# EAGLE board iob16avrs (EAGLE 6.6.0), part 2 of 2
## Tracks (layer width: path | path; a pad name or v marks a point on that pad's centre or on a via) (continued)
GND  (via drill 0.38) (continued)
  Top 0.254: 23.74,28.91 23.7,28.87 23.7,28.3 23.74,28.26 24.49,28.26 CF1.15 | 23.74,28.91 CF1.39 | 23.74,28.91 23.7,29.02 23.7,29.51 23.74,29.55 24.49,29.55 CF1.14 26.43,29.55 v27.04,29.55 | IC12.110 87.69,56.53 86.89,56.53 86.86,56.57 86.86,56.98 86.89,57.02 87.69,57.02 IC12.109 89.26,57.02 v89.87,57.02 | v87.05,40.03 87.69,40.03 IC12.143 | v93.83,39.08 93.83,38.47 IC12.8 | v87.05,44.03 87.69,44.03 IC12.135 | v89.87,47.54 89.26,47.54 IC12.128 | v98.32,39.08 98.32,38.47 IC12.17 | v87.05,52.03 87.69,52.03 IC12.119 | v102.32,39.08 102.32,38.47 IC12.25 | v106.32,39.08 106.32,38.47 IC12.33 | v91.35,57.48 91.35,58.09 IC12.106 | v95.35,57.48 95.35,58.09 IC12.98 | v108.27,43.54 108.92,43.54 IC12.45 | v108.27,47.04 108.92,47.04 IC12.52 | v99.85,57.48 99.85,58.09 IC12.89 | v103.85,57.48 103.85,58.09 IC12.81 | v108.27,51.54 108.92,51.54 IC12.61 | v107.85,60.26 107.85,59.65 IC12.73 | v23.84,14.92 24.49,14.92 CF1.50 | v23.84,25.74 24.49,25.74 CF1.17 | v23.84,27 CF1.16 | v23.84,32.07 24.49,32.07 CF1.12 | v23.84,33.36 24.49,33.36 CF1.11 | v23.84,34.62 CF1.10 | v23.84,37.17 24.49,37.17 CF1.8 | v23.84,46.05 CF1.1 | v34.16,71.77 34.81,71.77 IC8.1 | v61.79,70.09 62.43,70.09 IC9.19 | IC17.7 v129.95,7.65 | v129.95,17.82 130.59,17.82 IC15.7 | v136.08,14.01 136.73,14.01 IC17.13 | v129.95,20.33 130.59,20.33 IC15.5 | v136.08,19.08 IC15.9 | v136.08,21.63 136.73,21.63 IC15.11 | v126.71,32.41 IC13.10 | v136.08,24.14 136.73,24.14 IC15.13 | v136.77,42.58 137.41,42.58 IC13.19 | v120.65,60.11 121.3,60.11 IC11.8 | v9.32,72.3 9.32,72.95 C8.2 7.19,75.53 IC1.27 | v24.9,79.39 25.55,79.39 IC2.16 | v28.37,74.85 28.37,75.5 C5.2 28.19,76.36 27.36,77.19 17.19,77.19 17.19,78.69 IC1.47 17.19,78.86 16.69,78.86 IC1.46
  Top 0.254: v48.18,66.93 48.83,66.93 C14.2 | v43.95,79.39 44.6,79.39 IC3.16 | v125.11,15.61 125.11,15 IC16.4 | v63,79.39 63.65,79.39 IC4.16 | v69.86,74.97 69.86,75.62 C6.2 | v93.26,66.55 IC7.8 | v83.35,79.39 84,79.39 IC5.16 | v89.87,75.01 90.51,75.01 C9.2 | v101.1,84.49 101.75,84.49 REG2.5.2 | v101.1,85.75 REG2.5.1 | v104.91,89.75 104.91,89.14 C3.2 | v109.98,84.49 110.63,84.49 REG3.3.2 | REG3.3.1 v109.98,85.75 | v113.72,86.78 113.72,87.43 C4.2 | v134.06,67.31 134.71,67.31 C10.2 | v110.36,34.62 111.01,34.62 R7.1 | v114.13,67.04 114.13,67.69 X1.P$2 | v134.18,63.31 134.82,63.31 C11.2 | v18.47,57.33 18.47,57.98 R4.2 | v105.45,96.46 105.45,97.1 C1.- | v114.33,96.46 C2.- | v19.34,61.86 19.99,61.86 IC10.7 | v34.16,60.34 34.81,60.34 IC8.10 | v51.73,59.96 52.37,59.96 IC9.10 | v29.55,71.35 30.2,71.35 C13.2 | v107.45,77.65 108.28,77.64 C7.2 | v79.43,66.4 80,66.4 IC6.8 | v59.73,37.48 59.73,36.91 C17.2 | v55.92,25.67 56.53,25.67 IC14.8
  Bottom 0.254: C106.2 113.91,49.59 113.91,48.83 113.87,48.79 113.87,47.96 C102.2 113.87,46.47 v113.87,45.82 | C103.2 84.38,49.75 84.38,48.68 C104.2 84.38,47.19 v84.38,46.55 | C107.2 98.97,63.12 98.55,63.12 98.51,63.16 98.02,63.16 C105.2 96.53,63.16 v95.89,63.16 | C100.2 98.55,33.48 97.6,33.48 C101.2 96.15,33.48 v95.5,33.48
  pour GND$: 0,0 157.53,0 157.53,106.73 0,106.73
HS  (via drill 0.38)
  Top 0.178: v69.14,47.96 69.81,47.28 77.95,47.28 83.69,53.02 87.69,53.02 IC12.117 | v70.24,74.02 71.88,75.65 v77.09,75.65 | v87.16,87.85 88.3,88.99 99.31,88.99 104.08,93.75 135.24,93.75 140.04,88.95 146.1,88.95 146.94,89.79 149.19,89.79 VGA.13
  Bottom 0.178: v69.14,47.96 69.44,48.26 69.44,66.89 70.24,67.69 v70.24,74.02 | v77.09,75.65 82.74,81.31 82.74,83.43 v87.16,87.85
INTGNT_L  (via drill 0.38)
  Top 0.178: v83.92,42.35 83.92,41.44 84.46,40.91 86.66,40.91 86.74,40.98 87.69,40.98 IC12.141 | v81.1,55.42 80.76,55.77 74.36,55.77 SBC.10
  Bottom 0.178: v83.92,42.35 83.31,42.96 83.31,53.21 v81.1,55.42
INTREQ_L  (via drill 0.38)
  Top 0.178: v96.11,60.26 96.27,60.26 96.27,59.65 IC12.96 | v88.19,57.75 87.58,58.36 83.96,58.36 82.68,57.08 72.73,57.08 71.84,56.18 SBC.9
  Route2 0.178: v96.11,60.26 93.14,57.29 93.14,57.25 92.72,56.83 90.97,56.83 90.06,57.75 v88.19,57.75
IOCLR_L  (via drill 0.38)
  Top 0.178: v60.6,99.09 59.27,100.42 12.26,100.42 12.26,98.82 IC1.12 | v100.89,60.26 100.84,60.26 100.84,59.65 IC12.87
  Route2 0.178: v100.89,60.26 99.66,60.26 94.28,54.89 90.78,54.89 90.13,55.54 83.96,55.54 81.83,53.4 74.36,53.4 SBC.12
  Bottom 0.178: v60.6,99.09 60.53,99.01 60.53,96.3 64.34,92.49 70.47,92.49 70.47,82.32 70.74,82.05 70.74,74.6 72.96,72.54 72.96,66.96 72.63,66.63 72.63,54.74 73.32,54.05 SBC.12
KB_CLK  (via drill 0.38)
  Top 0.178: v84.72,41.55 85.64,42.47 87.69,42.47 IC12.138 | v81.52,19 81.71,18.81 114.4,18.81 119.7,24.1 v124.23,24.1
  Bottom 0.178: v84.72,41.55 82.32,39.15 82.32,25.4 81.52,24.6 v81.52,19 | v124.23,24.1 139.24,39.12 139.24,55.23 146.05,62.04 146.05,68.76 146.74,69.47 KBD.6
KB_DATA  (via drill 0.38)
  Top 0.178: v90.02,44.11 90.02,44.34 89.41,44.95 89.26,44.95 IC12.133 | v82.97,37.06 84.57,35.46 v87.69,35.46 | v88.72,30.66 v106.48,30.66 | v110.63,32.37 v118.25,32.37 | v117.45,36.22 118.14,36.91 129.49,36.91 v130.75,38.16 | v136.77,45.82 142.6,51.65 142.6,58.81 144.96,58.81 148.92,62.78 148.92,67.04 149.26,67.04 KBD.1
  Route2 0.178: v82.97,37.06 v90.02,44.11 | v106.48,30.66 106.9,30.66 107.96,31.72 109.98,31.72 v110.63,32.37
  Bottom 0.178: v87.69,35.46 88.72,34.43 v88.72,30.66 | v118.25,32.37 117.72,32.91 117.72,35.95 v117.45,36.22 | v130.75,38.16 136.77,44.18 v136.77,45.82
LOAD_DAR_H  (via drill 0.38)
  Top 0.178: v47.46,59.92 46.96,59.92 46.85,60.03 IC8.11 | v49.14,49.21 49.75,48.6 70.47,48.6 SBC.15
  Bottom 0.178: v47.46,59.92 49.14,58.24 v49.14,49.21
LXDAR_L  (via drill 0.38)
  Top 0.178: v72.45,41.21 72.45,40.91 72.53,40.84 72.53,37.86 73.37,37.02 73.71,37.01 75.39,35.31 78.78,35.31 79.65,34.43 98.78,34.43 98.78,36.91 IC12.18
  Bottom 0.178: v72.45,41.21 72.68,41.44 72.68,49.4 73.41,50.13 SBC.14
MA0  (via drill 0.38)
  Top 0.178: v15.27,95.89 15.27,97.26 IC1.6 | v20.71,90.44 21.02,90.13 37.82,90.13 38.13,89.83 38.35,89.83 IC2.25 40.53,89.83 40.56,89.87 44.22,89.87 44.49,90.13 55.54,90.13 v55.8,89.9 56.07,89.64 56.6,89.64 56.68,89.56 IC3.25 59.58,89.83 59.61,89.87 62.51,89.87 62.81,90.17 66.13,90.17 66.51,89.79 76.45,89.79 IC4.25 78.63,89.79 78.82,89.79 79.16,90.13 96.49,90.13 96.8,89.83 IC5.25 | v63,40.94 69.48,34.47 72.17,34.47 72.17,32.39 73.37,31.19 SBC.30
  Bottom 0.178: v20.71,90.44 v15.27,95.89 | v63,40.94 61.02,42.93 61.02,46.13 59.46,47.69 59.46,88.61 57.21,90.86 55.8,90.86 v55.8,89.9
MA1  (via drill 0.38)
  Top 0.178: v28.37,99.09 27.42,100.04 14.77,100.04 14.77,98.82 IC1.7 | v32.41,87.12 38.35,87.12 IC2.23 40.53,87.31 40.56,87.35 44.26,87.35 44.49,87.58 53.14,87.58 53.4,87.31 57.4,87.31 IC3.23 59.58,87.27 59.61,87.31 63.08,87.31 | 63.08,87.31 63.23,87.31 63.35,87.43 63.39,87.43 63.39,87.46 63.42,87.46 63.42,87.5 63.46,87.5 63.46,87.54 63.5,87.54 63.5,87.58 63.54,87.58 63.54,87.62 65.94,87.62 66.28,87.27 76.45,87.27 IC4.23 78.63,87.31 78.85,87.31 79.12,87.58 86.28,87.58 86.66,87.2 96.8,87.2 IC5.23 | v66.32,31.99 68.81,29.5 71.74,29.5 72.99,28.26 SBC.32 | v63.08,87.35 63.08,87.31
  Bottom 0.178: v28.37,99.09 29.36,98.09 32.41,98.09 v32.41,87.12 | v66.32,31.99 64.91,33.4 64.91,57.4 63.65,58.66 63.65,86.78 v63.08,87.35
MA2  (via drill 0.38)
  Top 0.178: v28.22,94.06 14.27,94.06 14.27,97.26 IC1.8 | v30.81,91.47 31.19,91.08 38.35,91.08 IC2.26 40.53,91.08 41.06,91.08 41.4,91.43 46.89,91.43 47.19,91.12 57.37,91.12 57.4,91.08 IC3.26 59.58,91.08 61.82,91.08 62.17,91.43 65.94,91.43 66.24,91.12 68.26,91.12 | 68.26,91.12 76.42,91.12 76.45,91.08 IC4.26 78.63,91.08 78.85,91.08 79.2,91.43 96.49,91.43 96.8,91.12 IC5.26 | v68.38,37.63 69.06,36.94 72.17,36.94 72.17,35 73.41,33.74 SBC.28 | v68.26,90.82 68.26,91.12
  Bottom 0.178: v30.81,91.47 v28.22,94.06 | v68.38,37.63 68.26,37.74 v68.26,90.82
MA3  (via drill 0.38)
  Top 0.178: v9.44,96.65 9.28,96.65 9.28,97.26 IC1.18 | v11.84,93.94 13.06,92.72 37.78,92.72 38.16,92.34 38.35,92.34 IC2.27 40.53,92.38 41.29,92.38 41.59,92.68 46.89,92.68 47.16,92.42 57.33,92.42 57.4,92.34 IC3.27 59.58,92.11 61.02,92.11 61.6,92.68 62.36,92.68 | 62.36,92.68 65.94,92.68 66.21,92.42 76.38,92.42 76.45,92.34 IC4.27 78.63,92.38 78.89,92.38 79.2,92.68 96.49,92.68 96.8,92.38 IC5.27 | v63,47.23 70.72,39.52 71.34,39.52 72.01,38.85 72.17,38.66 72.17,37.45 73.37,36.26 SBC.26 | 62.36,92.68 v62.36,92.46
  Bottom 0.178: v9.44,96.65 11.84,94.25 v11.84,93.94 | v63,47.23 62.43,47.8 62.43,79.04 62.36,79.12 v62.36,92.46
MA4  (via drill 0.38)
  Top 0.178: IC5.5 84,93.1 83.96,93.07 79.04,93.07 78.78,92.8 68.11,92.8 67.81,93.1 65.82,93.1 IC4.5 63.65,93.1 61.1,93.1 v60.76,92.76 60.38,92.8 57.29,92.8 57.06,93.03 46.85,93.03 46.77,93.1 IC3.5 44.6,93.1 41.48,93.1 41.17,92.8 38.24,92.8 37.94,93.1 27.72,93.1 IC2.5 25.55,93.64 14.12,93.64 13.17,94.59 8.79,94.59 8.79,97.26 IC1.19 | v62.01,45.67 63.23,45.67 70.47,38.43 SBC.23
  Bottom 0.178: v62.01,45.67 59.84,47.84 59.84,91.85 v60.76,92.76
MA5  (via drill 0.38)
  Top 0.178: 67.61,91.5 66.4,91.5 66.05,91.85 65.82,91.85 IC4.6 63.69,91.81 62.01,91.81 61.71,91.5 57.29,91.5 56.98,91.81 46.81,91.81 46.77,91.85 IC3.6 44.6,91.85 41.29,91.85 40.94,91.5 38.16,91.5 37.55,92.11 27.72,92.11 IC2.6 25.55,92.34 5.63,92.34 5.63,98.78 6.88,100.04 8.14,100.04 8.14,98.82 IC1.20 | 67.61,91.5 78.74,91.5 79.04,91.81 84,91.81 IC5.6 | v68.38,36.49 69.9,36.49 70.47,35.92 SBC.25 | 67.61,91.5 v67.61,91.77
  Bottom 0.178: v68.38,36.49 67.61,37.25 v67.61,91.77
MA6  (via drill 0.38)
  Top 0.178: v7.76,96.65 7.76,97.26 IC1.21 | v10.96,91.69 11.57,91.08 25.55,91.08 IC2.7 27.72,90.55 27.76,90.51 37.97,90.51 38.24,90.25 44.07,90.25 44.41,90.59 44.6,90.59 IC3.7 46.77,90.55 56.98,90.55 57.16,90.38 | 57.16,90.38 57.29,90.25 62.36,90.25 62.7,90.59 63.65,90.59 IC4.7 65.82,90.55 66.28,90.55 66.66,90.17 78.66,90.17 79.01,90.51 83.96,90.51 84,90.55 IC5.7 | v63,39.12 68.07,34.05 69.79,34.05 70.47,33.36 SBC.27 | v56.95,90.21 57.06,90.32 57.1,90.32 57.16,90.38
  Bottom 0.178: v7.76,96.65 8.98,95.43 8.98,93.68 v10.96,91.69 | v63,39.12 60.64,41.48 60.64,45.97 58.36,48.26 58.36,68.49 57.59,69.25 57.59,89.56 v56.95,90.21
MA7  (via drill 0.38)
  Top 0.178: v7.26,99.39 7.26,98.82 IC1.22 | v19.53,90.44 20.22,89.75 25.55,89.75 IC2.8 27.72,89.37 37.86,89.37 38.24,88.99 44.07,88.99 44.37,89.29 44.6,89.29 IC3.8 46.77,89.29 46.81,89.26 56.45,89.26 56.72,88.99 59.73,88.99 60.03,89.29 63.08,89.29 | 63.08,89.29 63.65,89.29 IC4.8 65.82,89.29 66.05,89.29 66.36,88.99 78.78,88.99 79.04,89.26 83.96,89.26 84,89.29 IC5.8 | v65.82,33.4 67.88,33.4 70.47,30.81 SBC.29 | v63.08,89.52 63.08,89.29
  Bottom 0.178: v7.26,99.39 9.32,97.33 14.62,97.33 14.62,95.35 v19.53,90.44 | v65.82,33.4 65.71,33.52 65.71,68.99 64.03,70.66 64.03,88.57 v63.08,89.52
MA8  (via drill 0.38)
  Top 0.178: v9.63,93.94 8.9,93.94 6.92,95.92 6.77,95.92 6.77,97.26 IC1.23 | v11.84,88.53 25.55,88.53 IC2.9 27.72,88.04 27.99,87.77 38.16,87.77 38.24,87.69 41.1,87.69 41.44,88.04 44.6,88.04 IC3.9 46.77,88 53.63,88 v53.67,87.96 53.98,87.73 59.73,87.73 59.99,88 63.65,88 IC4.9 65.82,88.04 66.05,88.04 66.4,87.69 78.74,87.69 79.04,88 84,88 IC5.9 | v54.24,28.45 56.34,26.35 69.18,26.35 70.47,27.65 SBC.31
  Bottom 0.178: v9.63,93.94 11.84,91.73 v11.84,88.53 | v54.24,28.45 53.52,29.17 53.52,36.41 54.32,37.21 54.32,53.29 53.59,54.01 53.59,85.79 53.67,85.86 v53.67,87.96
MA9  (via drill 0.38)
  Top 0.178: 53.02,24.6 69.98,24.6 70.47,25.1 SBC.33 | 53.02,24.6 26.43,24.6 CF1.18 | v6.27,95.5 6.27,97.26 IC1.24 | v6.92,91.69 11.34,87.27 25.55,87.27 IC2.10 27.72,86.74 28.03,86.44 44.26,86.44 44.6,86.78 IC3.10 46.77,86.74 47.08,86.44 53.02,86.44 | 53.02,86.44 59.69,86.44 59.96,86.7 63.58,86.7 63.65,86.78 IC4.10 65.82,86.74 70.66,86.74 70.97,86.44 83.69,86.44 84,86.74 IC5.10 | 53.02,24.6 v53.02,24.71 | v53.02,86.13 53.02,86.44
  Bottom 0.178: v6.27,95.5 6.92,94.86 v6.92,91.69 | v53.02,24.71 v53.02,86.13
MA10
  Top 0.178: IC5.11 84,85.48 83.96,85.45 79.04,85.45 78.7,85.1 66.43,85.1 66.05,85.48 65.82,85.48 IC4.11 63.65,85.48 60.45,85.48 60.15,85.18 57.29,85.18 56.98,85.48 46.77,85.48 IC3.11 44.6,85.48 41.4,85.48 41.02,85.1 37.17,85.1 36.79,85.48 27.72,85.48 IC2.11 25.55,85.48 6.27,85.48 6.27,79.62 IC1.25 6.08,78.05 3.04,78.05 3.04,44.64 24.33,23.34 24.49,23.34 CF1.19 26.43,23.34 47.99,23.34 48.72,24.07 67.08,24.07 70.47,20.68 SBC.37
MA11  (via drill 0.38)
  Top 0.178: 54.62,23.69 64.91,23.69 70.47,18.12 SBC.39 | 54.62,23.69 48.87,23.69 47.23,22.05 26.43,22.05 CF1.20 | IC5.12 84,84.23 79.54,84.23 79.2,83.88 76.34,83.88 76.04,84.19 65.86,84.19 65.82,84.23 IC4.12 63.65,84.23 v60.64,84.23 | v15.57,80.23 15.65,80.23 15.99,79.88 16.14,79.88 16.14,79.62 IC1.45 | v19.8,84.46 25.55,84.46 IC2.12 27.72,84.23 27.95,84.23 28.3,83.88 40.64,83.88 40.94,84.19 44.56,84.19 44.6,84.23 IC3.12 46.77,84.46 v55.69,84.46 | 54.62,23.69 v54.62,23.42
  Route2 0.178: v60.64,84.23 58.01,84.23 57.1,85.14 56.38,85.14 v55.69,84.46
  Bottom 0.178: v19.8,84.46 v15.57,80.23 | v54.62,23.42 54.89,23.69 54.89,64.8 54.28,65.41 54.28,82.85 55.54,84.11 v55.69,84.46
N$1  (via drill 0.38)
  Top 0.178: v108.31,53.98 108.92,53.98 IC12.66 | v124.23,43.76 124.23,43.23 124.88,42.58 127.36,42.58 IC13.2
  Route2 0.178: v108.31,53.98 110.1,53.98 117.64,46.43 121.68,46.43 124.23,43.88 v124.23,43.76
N$2
  Top 0.178: R8.1 60.72,17.89 60.34,17.89 BATA.+
N$3  (via drill 0.38)
  Top 0.178: v118.52,66.32 109.41,66.32 108.15,67.58 103.28,67.58 IC7.10 | v118.52,74.93 116.12,77.33 R1.1
  Bottom 0.178: J3.3 116.04,63.04 118.25,65.25 118.25,66.05 v118.52,66.32 v118.52,74.93
N$4  (via drill 0.38)
  Top 0.178: v117.14,52.6 110.48,52.6 IC12.63 | v117.07,44.6 117.41,44.26 122.82,44.26 123.85,43.23 123.85,42.85 124.08,42.85 124.8,42.13 126.82,42.13 127.36,41.59 IC13.3
  Bottom 0.178: v117.14,52.6 117.07,52.53 v117.07,44.6
N$5  (via drill 0.38)
  Top 0.178: v120.42,50.51 110.48,50.51 IC12.59 | v122.56,43.61 124.42,41.74 125.95,41.74 127.36,40.34 IC13.4
  Bottom 0.178: v120.42,50.51 122.56,48.37 v122.56,43.61
N$6  (via drill 0.38)
  Top 0.178: v130.75,44.07 125.64,49.17 111.93,49.17 111.85,49.1 110.48,49.1 IC12.56 | v130.75,39.8 129.98,39.04 129.34,39.04 IC13.5
  Bottom 0.178: v130.75,44.07 v130.75,39.8
N$7  (via drill 0.38)
  Top 0.178: v99.92,53.71 100.5,53.71 100.5,57.75 100.38,57.86 100.38,58.09 IC12.88 | v115.81,70.47 114.02,72.26 X1.P$3
  Route2 0.178: v99.92,53.71 99.92,55.38 103.09,58.55 103.09,61.6 103.47,61.98 104.31,61.98 105.37,60.91 108.12,60.91 v108.99,60.03
  Bottom 0.178: v108.99,60.03 111.54,60.03 111.54,66.21 v115.81,70.47
N$8
  Top 0.178: X2.1 124.23,12.1 124.23,12.87 124.12,12.87 IC16.3
N$10  (via drill 0.38)
  Top 0.178: v111.7,45.9 111.13,46.47 110.48,46.47 IC12.51 | v115.77,37.52 127.36,37.52 IC13.6
  Bottom 0.178: v111.7,45.9 115.13,42.47 115.13,38.16 v115.77,37.52
N$11
  Top 0.178: R11.1 61.44,43.5 60.34,43.5 BATB.+
N$15
  Top 0.178: IC12.43 110.48,42.55 114.02,42.55 117.91,46.43 127.47,46.43 132.04,41.86 132.04,36.53 129.34,36.53 IC13.7
N$16  (via drill 0.38)
  Top 0.178: v108.31,44.68 108.38,44.6 108.92,44.6 IC12.47 | v114.52,37.52 116.46,35.57 127.05,35.57 127.36,35.27 IC13.8
  Route2 0.178: v108.31,44.68 108.72,44.68 113.83,39.57 113.83,38.2 v114.52,37.52
N$17  (via drill 0.38)
  Top 0.178: v126.17,39.92 124.73,41.36 118.25,41.36 117.79,40.91 114.21,40.91 114.17,40.94 111.93,40.94 111.09,40.11 110.48,40.11 IC12.38 | v126.71,33.78 127.36,33.78 IC13.9
  Bottom 0.178: v126.17,39.92 125.91,39.65 125.91,34.58 v126.71,33.78
N$18  (via drill 0.38)
  Top 0.178: v104.04,36.33 103.89,36.33 103.89,36.91 IC12.28 | v105.94,33.25 106.17,33.02 v125.53,33.02 | v125.53,43.23 125.83,43.54 127.36,43.54 IC13.1
  Bottom 0.178: v104.04,36.33 104.31,36.07 104.31,34.89 v105.94,33.25 | v125.53,33.02 v125.53,43.23
N$19  (via drill 0.38)
  Top 0.178: v92.53,39.04 92.84,39.04 93.14,38.74 93.26,38.74 93.26,38.47 IC12.7 | v93.07,32.14 93.48,32.56 96.19,32.56 96.69,33.06 98.78,33.06 99.5,32.33 105.98,32.33 106.25,32.6 109.45,32.6 v109.68,32.37 | v110.82,19.84 111.54,20.56 115.62,20.56 119.81,24.75 129.03,24.75 130.59,23.19 IC15.3
  Bottom 0.178: v92.53,39.04 93.07,38.51 v93.07,32.14 | v109.68,32.37 109.49,32.18 109.49,21.17 v110.82,19.84
N$20  (via drill 0.38)
  Top 0.178: v94.21,36.33 94.4,36.53 94.78,36.53 94.78,36.91 IC12.10 | v94.86,27.38 95.12,27.65 v105.79,27.65 | v106.32,29.63 106.4,29.55 116.99,29.55 v117.07,29.63 | v119.16,27.53 120.95,25.74 130.59,25.74 IC15.1
  Bottom 0.178: v94.21,36.33 94.86,35.69 v94.86,27.38 | v105.79,27.65 106.32,28.18 v106.32,29.63 | v117.07,29.63 v119.16,27.53
N$21  (via drill 0.38)
  Top 0.178: v75.39,36.22 82.17,43 87.69,43 IC12.137 | v80.8,5.7 81.45,5.05 120.54,5.05 121.11,5.63 132.46,5.63 136.73,9.89 IC17.10
  Bottom 0.178: v75.39,36.22 75.32,36.18 75.32,28.19 73.56,26.43 72.68,26.43 72.68,14.85 73.66,13.87 75.65,13.87 75.65,10.85 v80.8,5.7
N$22  (via drill 0.38)
  Top 0.178: v90.02,53.75 98.78,53.75 98.78,58.09 IC12.91 | v84.61,17.17 85.48,16.29 104.99,16.29 107.2,14.08 112.12,14.08 112.57,13.63 112.57,12.48 112,11.91 112,10.31 129.76,10.31 130.59,11.15 IC17.4
  Route2 0.178: v90.02,53.75 86.78,53.75 76.3,43.27 76.3,36.49 76.04,36.22 76.04,25.74 v84.61,17.17
N$23  (via drill 0.38)
  Top 0.178: v69.06,42.09 74.7,42.09 83.58,50.97 87.69,50.97 IC12.121 | v69.41,5.44 71.46,3.38 v73.18,3.38 | v127.85,10.96 130.59,13.7 IC17.2
  Bottom 0.178: v69.06,42.09 69.02,42.05 69.02,36.22 68.15,35.34 67.69,35.34 67.69,16.14 69.41,14.43 v69.41,5.44 | v73.18,3.38 124.99,3.38 124.99,7.95 127.85,10.81 v127.85,10.96
N$24  (via drill 0.38)
  Top 0.178: v75.65,40.26 78.78,43.38 87.31,43.38 87.39,43.46 87.69,43.46 IC12.136 | v81.94,5.7 118.63,5.7 121.53,8.6 130.59,8.6 IC17.6
  Bottom 0.178: v75.65,40.26 76.04,39.88 76.04,11.61 v81.94,5.7
N$25  (via drill 0.38)
  Top 0.178: v89.87,49.63 89.83,49.59 89.26,49.59 IC12.124 | v98.67,4.03 99.31,4.67 120.69,4.67 121.26,5.25 134.63,5.25 136.73,7.34 IC17.8
  Route2 0.178: v89.87,49.63 88.34,49.63 85.98,47.27 84.19,47.27 77.33,40.41 77.33,26.31 81.52,22.12 81.52,21.17 90.21,12.48 90.67,12.48 91.69,11.46 91.69,11 92.72,9.97 93.18,9.97 94.25,8.9 94.25,8.45 v98.67,4.03
N$26  (via drill 0.38)
  Top 0.178: v142.9,39.8 140.58,39.8 139.4,40.98 IC13.18
  Bottom 0.178: v142.9,39.8 143.47,39.23 143.47,28.03 145.76,25.74 LPT.9
N$27  (via drill 0.38)
  Top 0.178: v145.99,37.33 144.16,39.15 139.97,39.15 139.4,39.73 IC13.17
  Bottom 0.178: v145.99,37.33 147.3,37.33 147.3,29.08 146.53,28.32 LPT.8
N$28  (via drill 0.38)
  Top 0.178: v144.12,36.56 141.91,38.77 139.4,38.77 IC13.16
  Bottom 0.178: v144.12,36.56 144.12,32.87 145.76,31.23 LPT.7
N$29
  Top 0.178: IC13.15 137.41,37.17 137.07,36.83 137.07,31.8 144.2,31.8 145.34,32.94 LPT.6
N$30
  Top 0.178: IC13.14 139.4,35.92 145.34,35.92 LPT.5
N$31
  Top 0.178: IC13.13 139.4,34.96 146.52,34.96 147.13,35.57 147.13,38.05 146.41,38.05 LPT.4
N$32  (via drill 0.38)
  Top 0.178: v144.77,34.32 139.74,34.32 139.4,33.97 IC13.12
  Bottom 0.178: v144.77,34.32 145.03,34.58 145.03,40.11 145.76,40.83 LPT.3
N$33  (via drill 0.38)
  Top 0.178: v140.68,33.59 140.27,33.59 139.4,32.72 IC13.11
  Bottom 0.178: v140.68,33.59 142.23,35.14 142.23,40.07 145.76,43.57 LPT.2
N$34  (via drill 0.38)
  Top 0.178: IC15.2 132.58,24.45 132.96,24.83 132.96,28.14 132.08,28.14 131.78,28.45 R9.1 131.78,30.01 131.78,32.6 137.26,38.09 140.61,38.09 v140.68,38.13
  Bottom 0.178: v140.68,38.13 140.68,41.24 145.76,46.32 LPT.1
N$35
  Top 0.178: 135.45,24.85 135.62,25.02 135.62,28.45 R10.1 | 135.45,24.85 132.54,21.93 IC15.4 | LPT.16 148.31,39.42 148.31,38.76 148.2,38.64 147.51,37.95 147.51,31.7 145.61,31.7 145.53,31.69 139.03,25.2 139.03,24.79 135.51,24.79 135.45,24.85
N$36
  Top 0.178: IC17.11 138.71,11.76 139.93,12.98 140.84,12.98 145.91,18.05 147.09,18.05 148.84,19.8 149.03,19.8 149.81,20.58 149.81,42.2 149.13,42.2 LPT.15
N$37
  Top 0.178: IC17.3 132.58,13.02 132.92,13.36 140.69,13.36 145.76,18.43 146.52,18.43 147.13,19.04 147.13,21.48 146.37,21.48 LPT.10
N$38
  Top 0.178: IC17.1 132.58,14.96 132.88,14.66 136.58,14.66 136.61,14.62 140.81,14.62 145.34,19.15 LPT.11
N$39
  Top 0.178: IC17.5 132.58,10.46 132.96,10.85 139.78,10.85 145.34,16.41 LPT.12
N$40
  Top 0.178: IC17.9 138.71,9.21 143.13,13.63 145.34,13.63 LPT.13
N$41  (via drill 0.38)
  Top 0.178: v85.26,45.78 86.09,45.78 86.78,46.47 87.69,46.47 IC12.130
  Bottom 0.178: v85.26,45.78 85.1,45.63 85.1,42.09 85.37,41.82 85.37,41.29 83.62,39.54 83.62,23.08 82.89,22.35 IO1.26
N$42  (via drill 0.38)
  Top 0.178: v83.96,44.03 83.73,44.36 83.73,46.85 86.86,49.97 87.69,49.97 IC12.123
  Route2 0.178: v83.96,44.03 83.96,43.84 77.71,37.59 77.71,27.42 82.47,22.66 83.65,22.66 84.38,21.93 IO1.24
N$43  (via drill 0.38)
  Top 0.178: v86.4,41.55 87.69,41.55 IC12.140
  Bottom 0.178: v86.4,41.55 86.4,23.3 87.35,22.35 IO1.22
N$44  (via drill 0.38)
  Top 0.178: v81.79,50.09 84.38,52.68 87.31,52.68 87.39,52.6 87.69,52.6 IC12.118
  Route2 0.178: v81.29,29.36 84.61,26.05 87.24,26.05 89.14,24.14 89.14,23.08 89.87,22.35 IO1.20
  Bottom 0.178: v81.79,50.09 81.56,49.86 81.56,29.63 v81.29,29.36
N$45  (via drill 0.38)
  Top 0.178: v127.5,50.81 125.15,50.81 125.15,53.9 123.39,55.65 120.99,55.65 120.99,55.99 116.19,60.8 114.48,60.8 113.26,62.01 106.9,62.01 106.9,59.65 IC12.75 | v124.84,29.63 124.19,28.98 98.59,28.98 97.64,28.03 v92.8,28.03
  Bottom 0.178: v127.5,50.81 127.36,50.7 127.36,32.14 v124.84,29.63 | v92.8,28.03 91.69,26.92 91.69,23.08 92.42,22.35 IO1.18
N$46  (via drill 0.38)
  Top 0.178: v114.48,41.55 110.48,41.55 IC12.41
  Route2 0.178: v114.48,41.55 118.1,37.94 118.1,34.39 112.15,28.45 110.9,28.45 107.66,25.21 107.54,25.21 106.48,24.14 106.48,23.69 105.45,22.66 96.72,22.66 96,21.93 IO1.16
N$47  (via drill 0.38)
  Top 0.178: v115.36,49.86 115.19,50.03 IC12.58 | v115.36,46.69 116.69,48.03 v121.86,48.03
  Route2 0.178: v121.86,48.03 123.36,48.03 126.19,45.19 126.19,40.86 125.36,40.03 125.36,35.53 116.03,26.19 112.36,26.19 111.53,25.36 111.53,21.19 110.86,20.53 98.86,20.53 97.86,21.53 IO1.14
  Bottom 0.178: v115.36,46.69 v115.36,49.86
N$48  (via drill 0.38)
  Top 0.178: v101.14,57.52 101.26,57.52 101.26,58.09 IC12.86 | v77.98,24.75 80.07,22.66 98.9,22.66 99.62,21.93 IO1.12
  Route2 0.178: v101.14,57.52 100.8,57.52 93.64,50.36 84.3,50.36 v77.44,43.5
  Bottom 0.178: v77.44,43.5 77.71,43.23 77.71,25.02 v77.98,24.75
N$49  (via drill 0.38)
  Top 0.178: v100.91,43.65 100.91,38.47 IC12.22
  Route2 0.178: v103.81,46.47 103.81,45.25 108.42,40.64 108.57,40.64 109.3,39.92 109.3,37.9 108.92,37.52 108.38,37.52 106.97,38.93 106.97,39.34 106.59,39.73 104.95,39.73 104.34,39.12 104.34,37.55 102.48,35.69 102.48,34.54 101.18,33.25 101.18,30.39 v101.83,29.74
  Bottom 0.178: v100.91,43.65 103.73,46.47 v103.81,46.47 | v101.83,29.74 101.87,29.71 101.87,23.08 102.59,22.35 IO1.10
N$50  (via drill 0.38)
  Top 0.178: v103.81,43.73 103.81,42.51 104.19,42.13 104.34,42.13 104.34,38.47 IC12.29
  Route2 0.178: v103.81,43.73 104.42,43.73 107.66,40.49 107.66,39.15 v108.65,38.16
  Bottom 0.178: v108.65,38.16 108.38,37.9 108.38,26.05 106.48,24.14 106.48,23.08 105.75,22.35 IO1.8
N$51  (via drill 0.38)
  Top 0.178: v112.57,44.11 110.71,45.97 110.48,45.97 IC12.50 | v112.65,25.51 111.54,24.41 111.54,22.66 109.45,22.66 108.72,21.93 IO1.6
  Bottom 0.178: v112.57,44.11 113.79,42.89 113.79,26.66 v112.65,25.51
N$52
  Top 0.178: R6.1 143.05,42.85 145.57,45.36 147.89,45.36 LPT.14
N$53  (via drill 0.38)
  Top 0.178: v114.55,43.99 110.59,47.96 110.48,47.96 IC12.54
  Route2 0.178: v114.55,43.99 114.55,43.69 117.64,40.6 117.64,39.88 118.33,39.19 118.67,39.19 119.05,38.81 119.05,34.81 112.31,28.07 112.23,28.07 109.49,25.32 109.49,23.08 110.21,22.35 IO1.4
N$54  (via drill 0.38)
  Top 0.178: v85.75,44.68 87.31,44.68 87.39,44.6 87.69,44.6 IC12.134 | v85.75,25.4 85.56,25.21 84.04,25.21 83.31,24.49 IO1.25
  Bottom 0.178: v85.75,44.68 85.75,29.32 86.02,29.06 86.02,25.67 v85.75,25.4
N$55  (via drill 0.38)
  Top 0.178: v82.66,52.91 84.3,54.55 87.69,54.55 IC12.114 | v84.65,39.65 v82.93,41.36
  Bottom 0.178: v82.66,52.91 82.93,52.64 v82.93,41.36 | v84.65,39.65 84.72,39.57 84.72,24.83 IO1.23
N$56  (via drill 0.38)
  Top 0.178: v90.02,42.05 89.26,42.05 IC12.139 | v90.28,25.55 89.94,25.21 89.1,25.21 88.38,24.49 IO1.21
  Bottom 0.178: v90.02,42.05 89.79,41.82 89.79,28.37 90.09,28.07 90.09,25.74 v90.28,25.55
N$57  (via drill 0.38)
  Top 0.178: v94.67,48.03 93.22,48.03 93.22,49.63 89.37,53.48 89.26,53.48 IC12.116
  Route2 0.178: v94.67,48.03 95.54,47.16 95.54,44.3 94.67,43.42 93.56,43.42 89.41,39.27 89.41,25.4 89.9,24.9 IO1.19
N$58  (via drill 0.38)
  Top 0.178: v93.87,49.71 99.24,49.71 106.82,57.29 107.28,57.29 107.28,58.09 IC12.74 | v82.97,26.39 83.31,26.05 86.02,26.05 86.63,25.44 86.63,23.11 91.27,23.11 92,23.84 IO1.17
  Route2 0.178: v93.87,49.71 91.12,49.71 87.77,46.36 87.77,45.29 87.16,44.68 86.66,44.68 84.99,43 83.65,43 79.77,39.12 79.77,31.27 79.73,31.23 79.73,29.63 v82.97,26.39
N$59  (via drill 0.38)
  Top 0.178: v106.36,51.46 107.89,52.98 108.92,52.98 IC12.64 | v107.73,27.27 106.74,26.28 103.54,26.28 101.41,24.14 101.41,23.11 96.72,23.11 96,23.84 IO1.15
  Route2 0.178: v106.36,43.61 106.74,43.61 113.18,37.17 113.41,37.17 113.79,36.79 113.79,33.32 v107.73,27.27
  Bottom 0.178: v106.36,51.46 106.44,51.38 106.44,43.69 v106.36,43.61
N$60  (via drill 0.38)
  Top 0.178: v122.25,42.01 122.06,41.82 120.19,41.82 120.19,42.85 119.16,43.88 115.89,43.88 114.1,42.09 110.48,42.09 IC12.42 | v122.29,34.28 122.25,34.32 117.11,34.32 v117.07,34.28
  Route2 0.178: v117.07,34.28 116.19,34.28 107.81,25.9 99.96,25.9 98.55,24.49 IO1.13
  Bottom 0.178: v122.25,42.01 122.29,41.97 v122.29,34.28
N$61  (via drill 0.38)
  Top 0.178: v102.21,53.71 102.29,53.71 102.29,58.09 IC12.84 | v93.18,25.74 93.71,25.21 98.9,25.21 99.62,24.49 IO1.11
  Route2 0.178: v94.09,42.77 94.09,42.16 91.08,39.15 91.08,37.9 89.79,36.6 89.79,29.13 v93.18,25.74
  Bottom 0.178: v102.21,53.71 100.57,53.71 100.57,49.78 95.05,44.26 95.05,43.73 v94.09,42.77
N$62  (via drill 0.38)
  Top 0.178: v103.73,61.33 103.73,60.95 103.24,60.45 102.9,60.45 102.9,59.65 IC12.83 | v113.03,55.92 114.4,54.55 119.01,54.55 124,49.56 127.24,49.56 133.07,43.73 133.07,34.43 132.38,34.43 126.17,28.22 109.6,28.22 107.28,25.9 105.03,25.9 103.62,24.49 IO1.9
  Route2 0.178: v103.73,61.33 103.73,60.34 105.68,58.39 110.55,58.39 v113.03,55.92
N$63  (via drill 0.38)
  Top 0.178: v106.1,41.14 106.13,41.1 108.92,41.1 IC12.40
  Route2 0.178: v106.1,41.14 105.79,41.14 v103.7,39.04
  Bottom 0.178: v103.7,39.04 103.39,38.74 103.39,33.78 105.14,32.03 105.14,24.9 IO1.7
N$64  (via drill 0.38)
  Top 0.178: v111.43,44.34 110.78,44.98 110.48,44.98 IC12.48 | v112.57,26.96 110.82,25.21 109.49,25.21 108.72,24.45 IO1.5
  Bottom 0.178: v111.43,44.34 112.84,42.93 112.84,37.13 112.5,36.79 112.5,27.04 v112.57,26.96
N$65  (via drill 0.38)
  Top 0.178: v115.58,53.25 115.35,53.48 110.48,53.48 IC12.65
  Route2 0.178: v115.58,53.25 123.28,45.55 124.5,45.55 124.88,45.17 124.88,39.92 112.65,27.69 112.38,27.69 110.82,26.12 110.82,24.9 IO1.3
N$66  (via drill 0.38)
  Top 0.178: v76.68,35.95 78.66,35.95 79.81,34.81 93.6,34.81 95.24,36.45 95.77,36.45 95.77,36.91 IC12.12 | v78.78,9.78 79.35,9.21 81.83,9.21 IO2.26
  Bottom 0.178: v76.68,35.95 76.95,35.69 76.95,11.61 v78.78,9.78
N$67  (via drill 0.38)
  Top 0.178: v92.11,36.33 92.27,36.33 92.27,36.91 IC12.5 | v92.42,29.74 92.3,29.63 v88.34,29.63
  Bottom 0.178: v92.11,36.33 92.42,36.03 v92.42,29.74 | v88.34,29.63 88.34,24.94 88.68,24.6 88.68,21.17 86.21,18.69 86.21,10.46 85.41,9.66 IO2.24
N$68  (via drill 0.38)
  Top 0.178: v138.48,68.26 139.01,68.26 139.05,68.22 RN2.8 | v140.31,89.6 144.54,93.83 VGA.1
  Bottom 0.178: v138.48,68.26 140.31,70.09 v140.31,89.6
N$69
  Top 0.178: RN2.7 140.92,67.01 141.61,66.32 146.33,66.32 148.96,68.95 148.96,70.89 150.86,72.8 150.86,91.24 148.62,91.24 147.78,92.08 145.49,92.08 VGA.2
N$70  (via drill 0.38)
  Top 0.178: v148.5,71.35 148.5,69.02 146.18,66.7 142.48,66.7 142.18,67.01 RN2.6
  Bottom 0.178: v148.5,71.35 144.58,75.27 144.58,83.73 145.8,84.95 145.8,88.53 145.07,89.26 VGA.3
N$71  (via drill 0.38)
  Top 0.178: v90.44,36.33 91.27,36.33 91.27,36.91 IC12.3
  Bottom 0.178: v90.44,36.33 90.47,36.3 90.47,26.28 91.24,25.51 91.24,13.97 88.68,11.42 88.68,10.39 87.96,9.66 IO2.22
N$72  (via drill 0.38)
  Top 0.178: v100.47,36.33 99.89,36.33 99.89,36.91 IC12.20 | v96.11,7.87 91.66,7.87 90.93,8.6 IO2.20
  Route2 0.178: v100.47,36.33 100.47,34.67 v98.13,32.33
  Bottom 0.178: v98.13,32.33 96.76,30.96 96.76,10.54 96.3,10.08 96.3,8.06 v96.11,7.87
N$73  (via drill 0.38)
  Top 0.178: v92.49,57.52 92.76,57.52 92.76,58.09 IC12.103
  Route2 0.178: v92.49,57.52 92.23,57.52 91.35,58.39 84,58.39 83.35,57.75 82.82,57.75 80.65,59.92 80.65,61.06 80.26,61.44 78.63,61.44 74.26,57.08 70.91,57.08 67.88,54.05 67.88,38.05 67.69,37.86 67.69,30.01 71.27,26.43 71.58,26.43 72.68,25.32 72.68,25.02 73.66,24.04 74,24.04 86.63,11.42 86.63,11 87.66,9.97 91.27,9.97 92,9.25 IO2.18
N$74  (via drill 0.38)
  Top 0.178: v88.07,62.09 97.79,62.09 97.79,59.65 IC12.93 | v76.38,52.76 v76.38,54.78
  Route2 0.178: v88.07,62.09 78.36,62.09 v76.45,60.19
  Bottom 0.178: v76.45,60.19 74.69,58.42 74.71,55.54 74.59,55.38 74.59,54.85 74.97,54.47 76.38,54.47 v76.38,54.78 | v76.38,52.76 74.85,51.23 74.85,47.31 76.8,45.36 76.8,36.75 77.33,36.22 77.33,12.14 84.15,5.32 94.63,5.32 94.63,8.52 IO2.16
N$75  (via drill 0.38)
  Top 0.178: v94.44,60.26 94.4,60.26 94.4,59.65 IC12.100
  Route2 0.178: v100.03,67.84 102.17,67.84 109.18,60.83 109.18,60.76 116.69,53.25 119.01,53.25 126.82,45.44 126.82,36.11 114.52,23.8 114.52,17.78 109.03,12.29 109.03,11.04 107.96,9.97 99.28,9.97 98.55,9.25 IO2.14
  Bottom 0.178: v94.44,60.26 94.86,60.68 94.86,63.58 95.92,64.64 98.28,64.64 99.28,65.75 100.03,66.51 v100.03,67.84
N$76  (via drill 0.38)
  Top 0.178: v130.75,59.16 131.36,59.16 IC11.16
  Bottom 0.178: v130.75,59.16 131.39,59.8 131.39,74.7 130.98,75.12 130.98,95.35 129.76,96.57 SER1.6
N$77  (via drill 0.38)
  Top 0.178: v80,60.8 80.65,61.44 96.42,61.44 96.95,60.91 97.26,60.91 97.26,59.65 IC12.94
  Route2 0.178: v80,60.8 73.73,54.52 73.42,54.52 72.32,53.42 72.32,42.94 71.04,41.67 70.74,41.67 69.02,39.95 69.02,35.38 v68.34,34.7
  Bottom 0.178: v68.34,34.7 68.64,34.39 68.64,16.33 70,14.97 70,9.91 71.11,8.8 72.3,8.8 72.3,5.05 73.25,4.1 98.02,4.1 98.02,6.16 100.04,8.18 IO2.12
N$78  (via drill 0.38)
  Top 0.178: v101.83,32.98 99.39,32.98 99.39,36.91 IC12.19
  Bottom 0.178: v101.83,32.98 104.38,30.43 104.38,18.47 104.61,18.24 104.61,12.1 103.92,11.42 103.92,10.39 103.2,9.66 IO2.10
N$79  (via drill 0.38)
  Top 0.178: v95.24,42.77 96.27,42.77 96.27,38.47 IC12.13 | v99.09,8.33 99.54,7.87 103.96,7.87 104.69,8.6 IO2.8
  Route2 0.178: v95.24,42.77 93.18,40.72 93.18,32.94 v97.41,28.71
  Bottom 0.178: v97.41,28.71 98.86,27.27 98.86,18.58 97.94,17.67 97.94,12.83 99.09,11.68 v99.09,8.33
N$80  (via drill 0.38)
  Top 0.178: v94.4,44.07 91.88,44.07 91.88,38.47 IC12.4 | v79.73,19.91 80,19.65 89.87,19.65 90.32,19.19 109.41,19.19 v109.68,19.46
  Route2 0.178: v94.4,44.07 94.4,44.45 95.16,45.21 95.16,47 94.78,47.38 90.86,47.38 87.69,44.22 87.69,43.76 85.37,41.44 85.37,41.29 v80.91,36.83
  Bottom 0.178: v80.91,36.83 80.53,36.45 80.53,32.56 79.73,31.76 v79.73,19.91 | v109.68,19.46 109.41,19.19 109.41,10.81 108.27,9.66 IO2.6
N$81  (via drill 0.38)
  Top 0.178: v91.16,35.46 92.76,35.46 92.76,36.91 IC12.6 | v95.12,13.09 96.76,11.46 96.76,9.97 109.07,9.97 109.79,9.25 IO2.4
  Route2 0.178: v91.16,35.46 91.16,33.86 91.12,33.82 91.12,31.95 93.83,29.25 93.83,14.39 v95.12,13.09
N$82
  Top 0.178: X2.2 122.21,12.1 122.21,12.87 122.29,12.87 IC16.2
N$83  (via drill 0.61)
  other vias: 120.68,6.38
N$85  (via drill 0.61)
  other vias: 125.76,6.38
N$86  (via drill 0.38)
  Top 0.178: v79.35,52.76 81.56,54.97 87.69,54.97 IC12.113
  Route2 0.178: v79.12,34.05 79.12,29.1 84.07,24.14 84.07,23.69 85.1,22.66 85.56,22.66 86.63,21.59 86.63,19.04 94.25,11.42 94.25,11 94.82,10.43 101.18,10.43 v101.56,10.81
  Bottom 0.178: v79.35,52.76 79.12,52.53 v79.12,34.05 | v101.56,10.81 101.41,10.96 101.41,14.62 101.18,14.85 101.18,16.45 101.87,17.13 CPREQ.2
N$91
  Top 0.178: IC10.3 21.97,67.27 27,72.3 27.03,72.35 27.03,72.36 32.69,72.36 32.72,72.34 32.72,72.3 33.9,71.12 52.37,71.12 IC9.1
N$92  (via drill 0.38)
  Top 0.178: v103.01,33.25 102.63,33.63 101.18,33.63 101.18,36.53 101.26,36.6 101.26,36.91 IC12.23 | v106.52,31.95 106.74,31.72 119.89,31.72 120.54,32.37 v121.3,32.37 | v120.78,62.04 121.09,62.36 121.3,62.36 IC11.6
  Route2 0.178: v103.01,33.25 104.31,33.25 105.6,31.95 v106.52,31.95
  Bottom 0.178: v121.3,32.37 123.2,34.28 123.2,59.61 v120.78,62.04
N$93  (via drill 0.38)
  Top 0.178: v95.53,39.19 95.36,39.19 95.36,37.69 IC12.11 | v113.19,48.53 113.36,48.69 124.53,48.69 v124.69,48.53 | v124.53,59.69 124.53,62.19 124.03,62.69 122.86,63.86 122.36,63.86 IC11.5
  Route2 0.178: v95.53,39.19 95.53,40.86 102.53,47.86 102.53,48.03 103.69,49.19 112.53,49.19 v113.19,48.53
  Bottom 0.178: v124.69,48.53 124.53,48.69 v124.53,59.69
N$94  (via drill 0.38)
  Top 0.178: v107.35,33.9 102.9,33.9 102.9,36.91 IC12.26 | v113.14,34.28 113.79,34.93 v126.56,34.93 | v126.82,64.95 123.28,64.95 IC11.4
  Route2 0.178: v107.35,33.9 112.76,33.9 v113.14,34.28
  Bottom 0.178: v126.56,34.93 126.82,35.19 v126.82,64.95
N$95  (via drill 0.38)
  Top 0.178: v100.19,39.04 100.27,39.04 100.27,38.47 IC12.21 | v101.18,28.33 101.45,28.6 125.64,28.6 v126.14,29.1 | v130.56,60.3 131.36,61.1 IC11.18
  Bottom 0.178: v100.19,39.04 102.48,36.75 102.48,34.54 101.18,33.25 v101.18,28.33 | v126.14,29.1 130.1,33.06 130.1,59.84 v130.56,60.3
N$96  (via drill 0.38)
  Top 0.178: v104.95,35.15 103.39,35.15 103.39,36.91 IC12.27 | v107.35,30.2 107.43,30.28 v126.4,30.28 | v130.75,66.47 IC11.22
  Bottom 0.178: v104.95,35.15 107.35,32.75 v107.35,30.2 | v126.4,30.28 129.72,33.59 129.72,65.44 v130.75,66.47
N$97  (via drill 0.38)
  Top 0.178: v85.71,53.9 85.79,53.98 87.69,53.98 IC12.115 | v87.31,64.6 88,65.29 89.83,65.29 91.73,67.2 108,67.2 109.64,65.56 v119.89,65.56 | v123.93,63.92 124.88,62.97 131.36,62.97 IC11.19
  Bottom 0.178: v85.71,53.9 86.06,54.24 86.06,63.35 v87.31,64.6 | v119.89,65.56 121.53,63.92 v123.93,63.92
N$101
  Top 0.178: IC11.10 123.28,57.29 125.53,55.04 125.53,52.98 C16.1
N$102
  Top 0.178: IC11.12 122.75,54.74 122.75,52.98 C16.2
N$103
  Top 0.178: IC11.13 133.34,54.74 134.79,54.74 C12.1
N$104
  Top 0.178: IC11.14 133.34,56.6 133.45,56.72 134.79,56.72 C12.2
N$105
  Top 0.178: IC11.11 121.3,56.6 120.92,56.98 120.92,58.2 123.39,58.2 128.65,52.95 C15.2
N$106
  Top 0.178: R4.1 14.88,59.92 11.38,63.42 6.35,63.42 5.44,64.34 SPKR.-
N$107
  Top 0.178: IC11.15 133.3,57.9 135.13,59.73 C11.1
N$110  (via drill 0.38)
  Top 0.178: v123.85,61.75 123.36,61.75 123.28,61.67 IC11.7
  Bottom 0.178: v123.85,61.75 125.76,63.65 125.76,83.43 126.75,84.42 SER2.3
N$112  (via drill 0.38)
  Top 0.178: IC11.3 v126.4,66.47
  Bottom 0.178: v126.4,66.47 126.59,66.66 126.59,74.85 SER3.3
N$113  (via drill 0.38)
  Top 0.178: v130.75,69.94 131.36,69.33 IC11.24
  Bottom 0.178: v130.75,69.94 130.56,70.13 130.56,93.18 129.72,94.02 SER1.5
N$114  (via drill 0.38)
  Top 0.178: v130.75,68.64 131.36,68.03 IC11.23
  Bottom 0.178: v130.75,68.64 128,71.39 128,93.22 127.2,94.02 SER1.3
R0  (via drill 0.38)
  Top 0.178: v89.87,54.89 93.64,54.89 93.64,56.68 94.78,57.82 94.78,58.09 IC12.99 | v101.75,63.69 101.83,63.61 120.23,63.61 121.18,64.57 126.29,64.57 126.56,64.3 130.98,64.3 131.2,64.53 139.05,64.53 RN2.1
  Bottom 0.178: v89.87,54.89 89.22,55.54 89.22,57.29 91.54,59.61 95.24,59.61 95.24,63.42 96.09,64.28 101.75,64.28 v101.75,63.69
RAM0_L  (via drill 0.38)
  Top 0.178: v55.96,31.34 56.22,31.34 56.53,31.04 IC14.4 | v56.15,58.09 56.68,58.62 v64.6,58.62 | v83.08,73.98 86.17,73.98 IC6.15
  Route2 0.178: v64.6,58.62 70.88,64.9 74,64.9 v83.08,73.98
  Bottom 0.178: v55.96,31.34 56.15,31.53 v56.15,58.09
RAM0_L_NV  (via drill 0.38)
  Top 0.178: v62.17,32.64 62.17,31.53 62.66,31.04 IC14.13 | v66.4,86.06 66.13,86.32 60.07,86.32 59.77,86.02 59.58,86.02 IC3.22
  Route2 0.178: v61.79,59.99 61.79,61.21 63.61,63.04 63.61,79.08 65.63,81.1 65.63,85.29 v66.4,86.06
  Bottom 0.178: v62.17,32.64 63.65,34.12 63.65,45.67 61.79,47.54 v61.79,59.99
RAM1_L  (via drill 0.38)
  Top 0.178: v53.67,37.48 53.52,37.48 53.52,32.79 56.53,29.78 IC14.5 | v83.24,72.64 84.11,71.77 86.17,71.77 IC6.13
  Route2 0.178: v53.67,37.48 53.67,38.89 56.15,41.36 56.15,48.22 64.07,56.15 64.38,56.15 70.75,62.52 71.55,62.52 72.69,63.67 72.69,63.96 73.29,64.55 75.14,64.55 v83.24,72.64
RAM1_L_NV  (via drill 0.38)
  Top 0.178: v37.13,45.97 39.23,45.97 43.15,42.05 57.56,42.05 63,36.6 65.02,36.6 65.02,30.16 64.64,29.78 IC14.12 | v37.78,85.75 38.35,85.75 IC2.22
  Bottom 0.178: v37.13,45.97 36.75,46.36 36.75,66.36 38.09,67.69 38.09,85.45 v37.78,85.75
RAM2_L  (via drill 0.38)
  Top 0.178: v60.03,31.27 60.03,30.01 58.51,28.49 IC14.6 | v63.92,51.16 64.87,52.11 76.64,52.11 v78.7,54.17 | v80.38,65.52 80.68,65.82 82.59,65.82 85.41,68.64 86.17,68.64 IC6.11
  Bottom 0.178: v60.03,31.27 60.91,31.27 61.63,31.99 64,31.99 64,51.08 v63.92,51.16 | v78.7,54.17 79.01,54.47 79.01,64.15 v80.38,65.52
RAM2_L_NV  (via drill 0.38)
  Top 0.178: v65.21,29.06 64.64,28.49 IC14.11 | v66.97,60.07 67.06,59.98 71.58,59.98 72.55,60.96 72.55,62.03 v74.52,62.03 | v99.54,85.56 98.93,85.56 IC5.22
  Bottom 0.178: v65.21,29.06 66.97,30.81 v66.97,60.07 | v74.52,62.03 76.99,64.49 76.99,74.05 88.49,85.56 v99.54,85.56
RAM3_L  (via drill 0.38)
  Top 0.178: v60.68,32.14 60.68,29.4 58.51,27.23 IC14.7 | v83.2,65.52 83.77,66.09 86.17,66.09 IC6.9
  Route2 0.178: v60.68,32.14 67.54,39 67.54,54.2 70.79,57.45 74.1,57.45 75.81,59.16 75.81,60.45 76.53,61.18 76.95,61.18 81.29,65.52 v83.2,65.52
RAM3_L_NV  (via drill 0.38)
  Top 0.178: v65.21,27.8 64.64,27.23 IC14.10 | v75.88,85.75 76.45,85.75 IC4.22
  Route2 0.178: v64.11,56.79 64.11,58.2 63.96,58.36 63.96,73.83 v75.88,85.75
  Bottom 0.178: v65.21,27.8 64.57,28.45 64.57,56.34 v64.11,56.79
RD_SR_L  (via drill 0.38)
  Top 0.178: v106.13,57.52 105.91,57.52 105.91,58.09 IC12.77 | v88.46,64.64 87.77,63.96 74.69,63.96 74.09,64.55 72.59,64.55 71.84,63.8 SBC.3
  Route2 0.178: v105.41,61.79 100,67.2 91.27,67.2 88.72,64.64 v88.46,64.64
  Bottom 0.178: v106.13,57.52 106.29,57.67 106.29,60.91 v105.41,61.79
READ_L  (via drill 0.38)
  Top 0.178: v17.17,64.11 19.72,66.66 19.72,67.92 19.99,67.92 IC10.2 | CF1.9 24.49,36.07 24.03,36.07 17.17,42.93 v17.17,49.21 17.55,49.37 22.39,54.2 54.24,54.2 | 54.24,54.2 69.94,54.2 70.47,53.67 SBC.11 | v105.45,60.26 105.41,60.26 105.41,59.65 IC12.78 | v101.07,86.7 99.77,88 98.93,88 IC5.24 | v16.98,72.3 12.64,76.64 7.66,76.64 7.66,77.71 7.66,77.8 7.66,78.03 IC1.28 | 54.36,88.84 56.38,88.84 56.64,88.57 57.4,88.57 IC3.24 59.58,88.57 59.8,88.57 60.07,88.84 65.98,88.84 66.17,88.65 76.38,88.65 76.45,88.57 IC4.24 78.63,88.57 78.85,88.57 79.12,88.84 87.24,88.84 v87.88,89.48 | 54.36,88.84 44.45,88.84 44.26,88.65 40.6,88.65 40.53,88.57 IC2.24 | v54.36,88.61 54.36,88.76 54.36,88.84 | 54.24,54.2 v54.24,54.28
  Bottom 0.178: v17.17,49.21 v17.17,64.11 17.02,64.49 17.02,72.26 v16.98,72.3 | v105.45,60.26 105.14,60.57 105.14,61.14 104.72,61.56 104.72,83.05 v101.07,86.7 100.91,87.08 100.84,87.16 100.84,91.05 100.46,91.43 87.88,91.43 v87.88,89.48 | v54.24,54.28 53.94,54.58 53.94,85.64 54.36,86.06 v54.36,88.61
RTC_RST  (via drill 0.38)
  Top 0.178: v86.7,57.71 86.44,57.71 86.44,56.41 87.24,55.61 87.69,55.61 IC12.112 | v100.09,64.92 100.08,64.91 v118.82,64.91 | v124.42,20.71 124.92,20.22 IC16.5
  Route2 0.178: v88.34,60.8 88.84,60.8 90.55,62.51 97.68,62.51 v100.09,64.92
  Bottom 0.178: v86.7,57.71 88.34,59.35 v88.34,60.8 | v118.82,64.91 123.58,60.15 123.58,21.55 v124.42,20.71
RTS2
  Top 0.178: IC11.21 133.34,65.37 141.03,65.37 141.3,65.1 141.3,61.9 142.06,61.9 HS2.2
S$2
  Bottom 0.178: 27.65,29.86 27.69,29.82
SKIP_L  (via drill 0.38)
  Top 0.178: v103.54,62.74 105.14,61.14 106.29,61.14 106.29,59.65 IC12.76 | v84.91,64.6 84.65,64.87 74.28,64.87 74.24,64.91 71.12,64.91 70,63.79 70,61.84 70.02,61.67 SBC.5
  Route2 0.178: v103.54,62.74 103.54,62.81 100.79,65.57 97.54,65.57 96.44,64.48 93.44,64.48 92.43,65.48 90.21,65.48 88.68,63.96 85.56,63.96 v84.91,64.6
SPEAKER
  Top 0.178: IC10.11 28.11,65.37 28.45,65.02 28.45,62.17 28.11,62.17 IC10.8 26.12,62.17 22.66,62.17 21.97,62.85 IC10.6 19.99,63.46 12.83,63.46 11.95,64.34 SPKR.+
SPKR  (via drill 0.38)
  Top 0.178: IC10.5 19.99,64.72 19.99,65.37 IC10.4 21.97,65.37 25.78,65.37 | IC10.9 26.16,63.46 26.16,64.11 IC10.10 26.12,64.72 25.78,65.06 25.78,65.37 | v90.78,60.8 90.89,60.91 96.38,60.91 96.72,60.57 96.76,60.57 96.76,59.65 IC12.95 | v89.48,59.5 89.41,59.42 89.26,59.42 89.19,59.36 74.53,59.36 74.37,59.51 70.56,59.51 70.48,59.43 70.48,59.42 70.32,59.27 38.62,59.27 36.91,60.99 33.78,60.99 28.11,66.66 IC10.12 | IC10.13 26.16,67.92 26.16,67.27 IC10.12 | 25.78,65.37 25.78,66.66 26.12,66.66 IC10.12
  Route2 0.178: v89.48,59.5 v90.78,60.8
STATUS_L  (via drill 0.38)
  Top 0.178: 98.51,75.43 96.08,75.43 IC7.1 | 98.51,75.43 99.85,75.43 100.84,74.43 101.1,74.43 IC7.15 | v83.46,68.22 82.25,68.22 81.98,67.96 81.94,67.88 IC6.7 | v87.02,76.37 87.95,77.29 97.56,77.29 98.51,76.34 98.51,75.5 98.51,75.43
  Bottom 0.178: v83.46,68.22 83.92,68.68 83.92,71.16 83.88,71.2 83.88,72.53 84.26,72.91 84.26,76.87 84.65,77.25 86.55,77.25 86.55,76.84 v87.02,76.37
TCK  (via drill 0.38)
  Top 0.178: v99.2,45.59 98.36,44.75 91.5,44.75 91.5,39.54 90.89,38.93 90.89,38.47 IC12.2
  Route2 0.178: v99.2,45.59 99.58,45.59 103.54,49.56 113.53,49.56 117.64,45.44 117.64,44.95 118.71,43.88 119.77,43.88 120.5,43.15 JTAG.4
TDI  (via drill 0.38)
  Top 0.178: v105.98,36.33 105.91,36.33 105.91,36.91 IC12.32 | v107.28,35.04 108.69,33.63 120.38,33.63 v120.42,33.67
  Bottom 0.178: v105.98,36.33 v107.28,35.04 | v120.42,33.67 120.92,34.16 120.92,39.57 JTAG.6
TDO  (via drill 0.38)
  Top 0.178: v115.77,38.81 107.12,38.81 107.05,38.74 106.9,38.74 106.9,38.47 IC12.34 | v115.77,41.55 116.76,42.55 117.94,42.55 JTAG.3
  Bottom 0.178: v115.77,38.81 v115.77,41.55
TMS  (via drill 0.38)
  Top 0.178: v99.35,46.74 97.75,45.14 91.12,45.14 91.12,42.24 89.48,40.6 89.26,40.6 IC12.142
  Route2 0.178: v99.35,46.74 99.35,48.22 103.89,52.76 106.17,52.76 108.88,55.46 112.27,55.46 v120.65,47.08
  Bottom 0.178: v120.65,47.08 120.92,46.81 120.92,46.13 JTAG.2
TX0  (via drill 0.38)
  Top 0.178: v128.65,73.41 123.28,68.03 IC11.2
  Bottom 0.178: v128.65,73.41 128.46,73.6 128.46,83.62 129.26,84.42 SER2.5
TX1
  Top 0.178: IC11.1 123.28,69.29 128.99,75.01 SER3.5
TX2  (via drill 0.38)
  Top 0.178: v125.11,63.92 131.36,63.92 IC11.20
  Bottom 0.178: v125.11,63.92 125.37,64.19 125.37,84.57 125.91,85.1 125.91,95.89 126.59,96.57 SER1.4
VBAT  (via drill 0.38)
  Top 0.178: v62.59,21.08 62.59,19.46 R8.2 62.25,19.8 64.19,17.86 64.51,17.56 65.24,16.83 65.86,16.86 66.03,16.69 | v59.08,29.97 59.08,32.98 58.51,32.98 IC14.2 58.51,33.59 58.78,33.59 v59.08,33.9 | v60.57,40.64 62.59,42.66 R11.2 | v121.03,17.48 121.03,18.05 IC16.8 | v116.27,9.66 112.8,6.2 90.67,6.2 v88.95,7.91 | v83.65,16.87 83.62,16.83 83.49,16.83 83.36,16.69 66.03,16.69 | 66.03,16.69
  Bottom 0.178: v62.59,21.08 59.08,24.59 v59.08,29.97 | v60.57,40.64 59.08,39.15 v59.08,33.9 | v121.03,17.48 116.27,12.71 v116.27,9.66 | v88.95,7.91 83.96,7.91 83.96,16.56 v83.65,16.87
VCC_NV  (via drill 0.38)
  Top 0.254: v79.27,98.44 78.63,98.44 IC4.32 | v86.78,98.44 96.8,98.44 IC5.32 | v89.14,75.69 89.14,74.7 89.87,73.98 90.47,73.98 90.51,73.94 C9.1 | v86.45,78.55 85.38,77.48 75.16,77.48 | 75.16,77.48 69.06,77.48 68.68,77.1 C6.1 67.54,75.62 66.24,74.32 44.37,74.32 v43.99,74.17 42.66,75.5 30.73,75.5 C5.1 | v75.16,77.83 75.16,77.6 75.16,77.48 | 56.15,34.24 56.15,32.68 56.53,32.3 IC14.3 | 56.15,34.24 56.53,34.24 IC14.1 | v48.18,65.9 48.79,65.9 48.83,65.86 C14.1 | v43.8,98.02 40.68,98.02 40.53,98.17 IC2.32 | v47.42,98.29 57.4,98.29 IC3.32 | v54.2,35.92 54.39,35.92 56.03,34.28 56.15,34.24
  Route2 0.254: v54.2,35.92 49.86,40.26 49.86,62.36 48.34,63.88 48.34,65.52 v48.18,65.9
  Bottom 0.254: v86.78,98.44 v79.27,98.44 78.89,98.29 77.29,96.69 75.16,96.69 v75.16,77.83 | v89.14,75.69 86.47,78.36 v86.45,78.55 | v48.18,65.9 43.99,70.09 v43.99,74.17 44.15,74.55 44.68,75.08 44.68,97.14 v43.8,98.02 44.07,98.29 v47.42,98.29
VCCO  (via drill 0.38, 0.61)
  Top 0.254: 119.16,81.92 119.16,81.64 119.43,81.64 | 90.32,56.53 90.55,56.76 90.55,58.09 | 90.32,56.53 89.87,56.07 89.26,56.07 IC12.111 | 90.55,58.09 90.44,58.09 IC12.108 | IC12.107 90.7,58.13 90.67,58.13 90.55,58.09 | v86.02,46.62 87.39,47.99 87.69,47.99 IC12.127 | v98.74,60.26 99.31,60.26 99.31,59.65 IC12.90 | 89.87,38.81 89.26,39.42 IC12.144 | 89.87,38.81 90.21,38.47 IC12.1 | 107.47,36.91 107.7,36.91 IC12.36 | 107.47,36.91 IC12.35 | 108.92,56.18 108.92,56.41 IC12.71 | 108.92,56.18 IC12.70 | v97.18,39.27 97.83,38.62 97.83,38.47 IC12.16 | v107.47,47.84 108.42,47.84 108.69,47.57 108.92,47.57 IC12.53 | v108.31,56.15 108.8,56.15 108.92,56.18 | v107.24,36.33 107.43,36.33 107.43,36.79 107.47,36.91 | 89.87,38.81 v90.44,39.38 | v90.67,56.22 90.63,56.22 90.32,56.53
  Top 0.61: REG3.3.6 119.43,83.21 119.43,83.19 | v119.43,80.42 119.43,81.64 119.43,83.19 | C2.+ 114.35,92 114.35,91.72 | REG2.5.4 102.86,81.92 104.67,81.92 104.67,83.21 | 104.67,83.21 REG2.5.3 | 104.67,83.21 105.21,83.74 105.21,86.46 106.5,87.02 106.76,87.99 106.76,88.25 C3.1 108.27,90.04 110.9,90.04 112.67,91.82 114.25,91.82 114.35,91.72 | 114.35,91.72 115.85,90.22 116.92,90.22 119.43,87.71 119.43,83.19 | REG3.3.5 116.95,81.92 119.16,81.92 119.38,81.92
  Route2 0.254: v107.47,47.84 107.81,47.99 108.34,48.53 v112.19,48.53 112.42,48.26 114.55,46.13 114.55,45.44 118.4,41.59 118.4,41.06 JTAG.5
  Bottom 0.254: 107.16,56.39 107.05,56.11 107.32,56.11 107.7,56.15 v108.31,56.15 | 91.14,48.22 90.89,48.22 | 107.32,47.84 v107.47,47.84 107.32,47.73 107.39,47.73 | C104.1 86.02,47.19 v86.02,46.62 86.17,46.28 86.44,46.01 86.44,45.29 86.86,44.87 88.95,44.87 88.95,45.52 89.6,46.16 91.14,46.16 | C107.1 99.01,60.8 99.01,60.53 v98.74,60.26 98.59,59.92 98.59,56.52 | 97.18,40.16 v97.18,39.27 97.03,38.93 97.03,35.84 C101.1 | 107.24,40.16 v107.24,36.33 | v112.19,48.53 112.19,47.96 C102.1 | v90.44,39.38 90.89,39.84 91.14,40.16 | 91.14,56.22 v90.67,56.22
  Bottom 0.61: v119.43,80.42 117.65,78.64 117.65,65.86 116.13,64.34 112.37,64.34 112.27,64.24 112.27,59.94 111.33,59 109.78,59 107.16,56.39
  Bottom 0.813: 91.19,56.52 98.59,56.52 107.32,56.52 107.32,56.11 107.32,47.84 107.32,47.73 107.32,40.16 107.24,40.16 97.18,40.16 91.14,40.16 91.14,46.16 91.14,48.22 91.14,56.22 91.14,56.52
VS  (via drill 0.38)
  Top 0.178: v92.38,55.54 93.26,55.54 93.26,58.09 IC12.102 | v101.03,62.81 101.03,64.34 108.61,64.34 v108.69,64.26 | v116.75,72.33 118.71,74.28 119.13,74.28 128.96,84.11 146.37,84.11 149.42,87.16 VGA.14
  Route2 0.178: v92.38,55.54 92.49,55.54 99.77,62.81 v101.03,62.81
  Bottom 0.178: v108.69,64.26 v116.75,72.33
WR_SR_L
  Top 0.178: IC12.101 93.79,59.65 93.79,60.15 77.41,60.15 74.36,63.2 SBC.4
WRITE_L  (via drill 0.38)
  Top 0.178: v27.04,32.87 26.43,32.87 CF1.36 | v42.58,50.51 70.47,50.51 SBC.13 71.84,50.55 72.7,49.69 75.71,49.69 v77.44,47.96 | v98.01,36.33 97.41,36.33 97.41,36.91 IC12.15 | v114.48,39.46 110.48,39.46 IC12.37 | v95.73,31.61 95.62,31.5 87.85,31.5 85.98,33.36 v78.47,33.36 | v12.9,99.39 12.79,99.39 12.79,98.82 IC1.11 | v29.51,95.73 30.62,94.63 38.35,94.63 IC2.29 40.53,94.93 40.83,95.24 46.93,95.24 47.23,94.93 57.4,94.93 IC3.29 59.58,94.93 59.61,94.97 63.31,94.97 63.54,95.2 66.01,95.2 66.28,94.93 76.45,94.93 IC4.29 78.63,94.93 78.85,94.93 79.12,95.2 96.53,95.2 96.8,94.93 IC5.29 98.93,94.36 99.24,94.36 99.24,91.73 v100.19,90.78
  Route2 0.178: v98.01,36.33 98.01,34.38 96.15,32.52 96.15,31.82 | 96.15,31.82 101.36,26.62 108,26.62 116.42,35.04 116.42,37.78 116.04,38.16 115.51,38.16 114.48,39.19 v114.48,39.46 | v95.73,31.61 96.08,31.79 96.15,31.82
  Bottom 0.178: v27.04,32.87 36.45,42.28 36.45,44.37 v42.58,50.51 | v78.47,33.36 78.09,33.74 78.09,47.31 v77.44,47.96 77.6,48.34 78.7,49.44 78.7,53.25 79.35,53.9 79.35,63.58 82.44,66.66 82.44,77.56 89.79,84.91 100.19,84.91 v100.19,90.78 | v12.9,99.39 17.67,99.39 18.05,99.77 27.72,99.77 27.72,97.52 v29.51,95.73
(copper drawn outside any net)
  shapes: Top area x1

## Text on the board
Top: Top | L1
Route2: Layer 2 | L2
GND$: Layer 3 | L3
Bottom: Bottom | L4
tPlace: Top Silk | 2 | 0 | 1 | 1 | 2 | -VT | RTS | CTS | -INIT
bPlace: Bot. Silk
tStop: Top Mask
bStop: Bot. Mask
Document: Material: FR2 | Thickness: 0.062" | Copper: 1 oz
_tplace: 2 | 2 | 6 | 6 | 1 | 1 | 11 | 11 | 1 | 1 | Female | Female | 10 | 10 | 2 | 2 | 1 | 1 | 5 | 5 | 10 | 10 | 10 | 10 | 15 | 15 | 2 | 2 | 1 | 1 | 10 | 10 | 6 | 6 | 3 | 3 | 1 | 1 | 2 | 2 | 1 | 1 | 2 | 2 | 8 | 8 | 5 | 5 | 3 | 3 | 2 | 2 | 1 | 1 | 14 | 14 | 1 | 1 | F25 | F25 | 1 | 1 | Lithium 3V | Lithium 3V | 1 | 1 | - | - | + | + | 6 | 6 | 50 | 50 | 1 | 1 | Lithium 3V | Lithium 3V | 26 | 26 | - | - | + | + | 1 | 1 | 13 | 13 | 25 | 25 | 26 | 26 | 2,54 | 2,54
